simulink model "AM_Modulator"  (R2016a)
settings: Solver=ode3  StartTime=0.0  StopTime=6  FixedStep=1/5000000  RelTol=1e-3

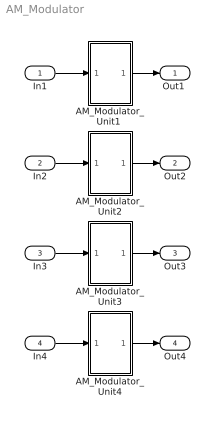
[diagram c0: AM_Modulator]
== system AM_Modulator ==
  In1 : Inport
  In2 : Inport  Port=2
  In3 : Inport  Port=3
  In4 : Inport  Port=4
  "AM_Modulator_Unit1 " : Subsystem
  AM_Modulator_Unit2 : Subsystem
  AM_Modulator_Unit3 : Subsystem
  AM_Modulator_Unit4 : Subsystem
  "Out1 " : Outport
  Out2 : Outport  Port=2
  Out3 : Outport  Port=3
  Out4 : Outport  Port=4
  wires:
  In1/1 -> "AM_Modulator_Unit1 "/1(In1)
  "AM_Modulator_Unit1 "/1(Out1) -> "Out1 "/1
  In2/1 -> AM_Modulator_Unit2/1(In1)
  AM_Modulator_Unit2/1(Out1) -> Out2/1
  In3/1 -> AM_Modulator_Unit3/1(In1)
  AM_Modulator_Unit3/1(Out1) -> Out3/1
  In4/1 -> AM_Modulator_Unit4/1(In1)
  AM_Modulator_Unit4/1(Out1) -> Out4/1

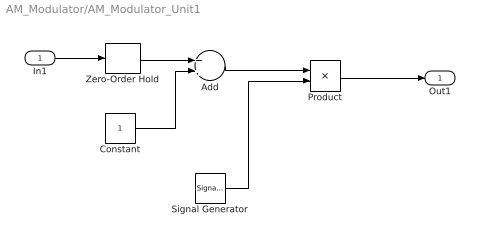
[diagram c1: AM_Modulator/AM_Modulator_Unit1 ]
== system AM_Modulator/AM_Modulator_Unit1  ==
  In1 : Inport
  Add : Sum
  Constant : Constant
  Product : Product
  Signal Generator : SignalGenerator  Frequency=500000
  Zero-Order Hold : ZeroOrderHold  SampleTime=0.0000002
  Out1 : Outport
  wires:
  Constant/1 -> Add/2
  Zero-Order Hold/1 -> Add/1
  Signal Generator/1 -> Product/2
  Product/1 -> Out1/1
  Add/1 -> Product/1
  In1/1 -> Zero-Order Hold/1

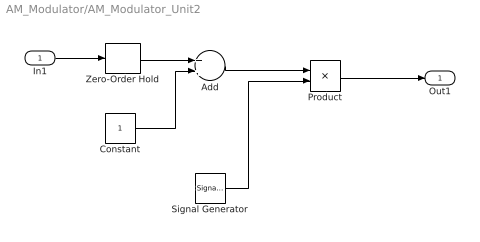
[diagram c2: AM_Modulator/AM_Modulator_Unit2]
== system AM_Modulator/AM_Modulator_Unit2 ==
  In1 : Inport
  Add : Sum
  Constant : Constant
  Product : Product
  Signal Generator : SignalGenerator  Frequency=500000
  Zero-Order Hold : ZeroOrderHold  SampleTime=0.0000002
  Out1 : Outport
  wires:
  Constant/1 -> Add/2
  Zero-Order Hold/1 -> Add/1
  Signal Generator/1 -> Product/2
  Product/1 -> Out1/1
  Add/1 -> Product/1
  In1/1 -> Zero-Order Hold/1

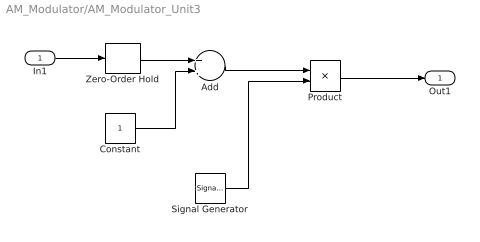
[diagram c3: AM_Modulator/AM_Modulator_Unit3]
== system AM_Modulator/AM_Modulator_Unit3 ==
  In1 : Inport
  Add : Sum
  Constant : Constant
  Product : Product
  Signal Generator : SignalGenerator  Frequency=500000
  Zero-Order Hold : ZeroOrderHold  SampleTime=0.0000002
  Out1 : Outport
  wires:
  Constant/1 -> Add/2
  Zero-Order Hold/1 -> Add/1
  Signal Generator/1 -> Product/2
  Product/1 -> Out1/1
  Add/1 -> Product/1
  In1/1 -> Zero-Order Hold/1

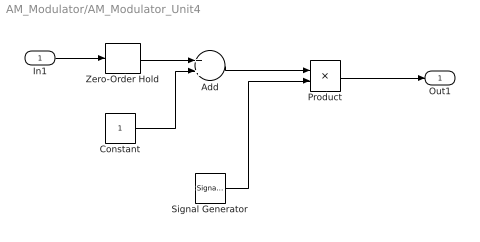
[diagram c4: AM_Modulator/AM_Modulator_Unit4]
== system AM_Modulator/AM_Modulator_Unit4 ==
  In1 : Inport
  Add : Sum
  Constant : Constant
  Product : Product
  Signal Generator : SignalGenerator  Frequency=500000
  Zero-Order Hold : ZeroOrderHold  SampleTime=0.0000002
  Out1 : Outport
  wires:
  Constant/1 -> Add/2
  Zero-Order Hold/1 -> Add/1
  Signal Generator/1 -> Product/2
  Product/1 -> Out1/1
  Add/1 -> Product/1
  In1/1 -> Zero-Order Hold/1
